(* Logix 5000 AddOnInstructionDefinition export Banner_Q5X_Jam_Param_v4; software revision 33.00; part 3 of 3 *)
(* tags used below, declared in another part *)
   Q5X : Banner_Q5X_Jam_v4;
   Port_Data : Banner_IOL_Port_v4;
   Port : DINT;
   Local_Control : DINT;
   Command_Being_Processed : BOOL;
   Update_Archive : BOOL;
   Index_Write_Inprocess : INT;
   Inprocess_Index : DINT;
(* Banner_Q5X_Jam_Param_v4, continued *)

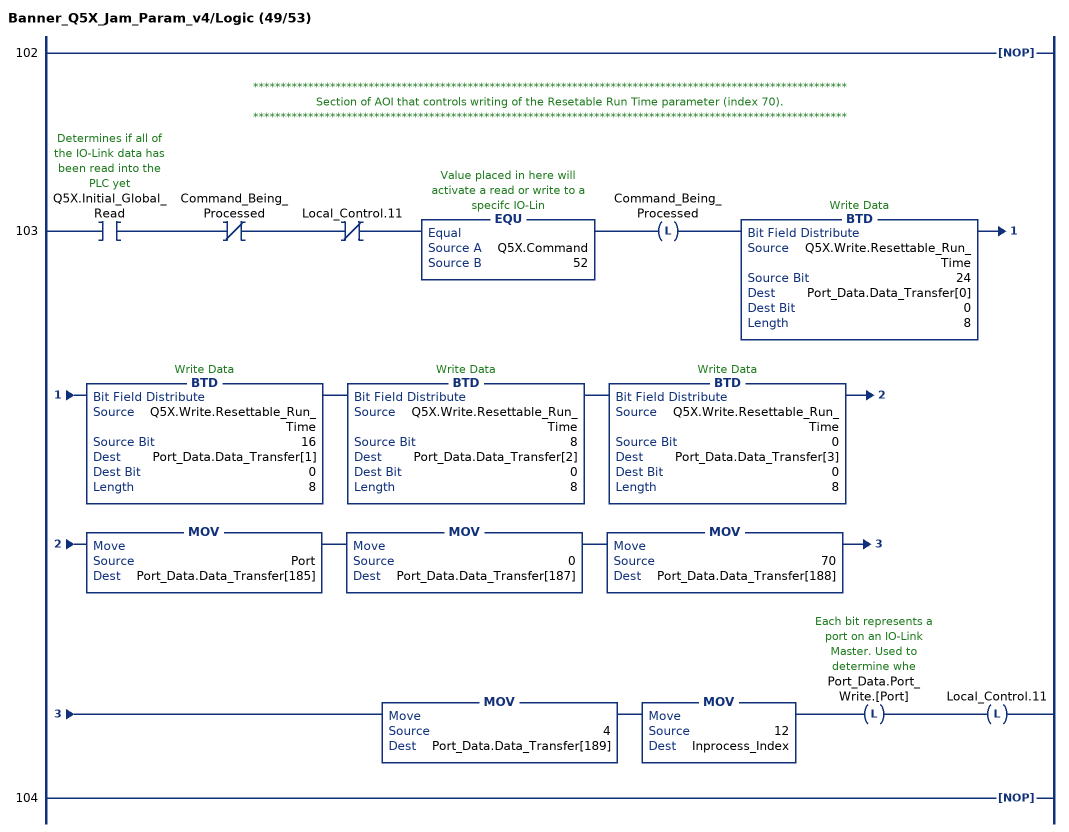
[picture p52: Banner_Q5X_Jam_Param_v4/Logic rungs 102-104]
   102: NOP();
   // ************************************************************************************************************
   // Section of AOI that controls writing of the Resetable Run Time parameter (index 70).
   // ************************************************************************************************************
   103: XIC(Q5X.Initial_Global_Read)XIO(Command_Being_Processed)XIO(Local_Control.11)EQU(Q5X.Command,52)OTL(Command_Being_Processed)BTD(Q5X.Write.Resettable_Run_Time,24,Port_Data.Data_Transfer[0],0,8)BTD(Q5X.Write.Resettable_Run_Time,16,Port_Data.Data_Transfer[1],0,8)BTD(Q5X.Write.Resettable_Run_Time,8,Port_Data.Data_Transfer[2],0,8)BTD(Q5X.Write.Resettable_Run_Time,0,Port_Data.Data_Transfer[3],0,8)MOV(Port,Port_Data.Data_Transfer[185])MOV(0,Port_Data.Data_Transfer[187])MOV(70,Port_Data.Data_Transfer[188])MOV(4,Port_Data.Data_Transfer[189])MOV(12,Inprocess_Index)OTL(Port_Data.Port_Write.[Port])OTL(Local_Control.11);
   104: NOP();
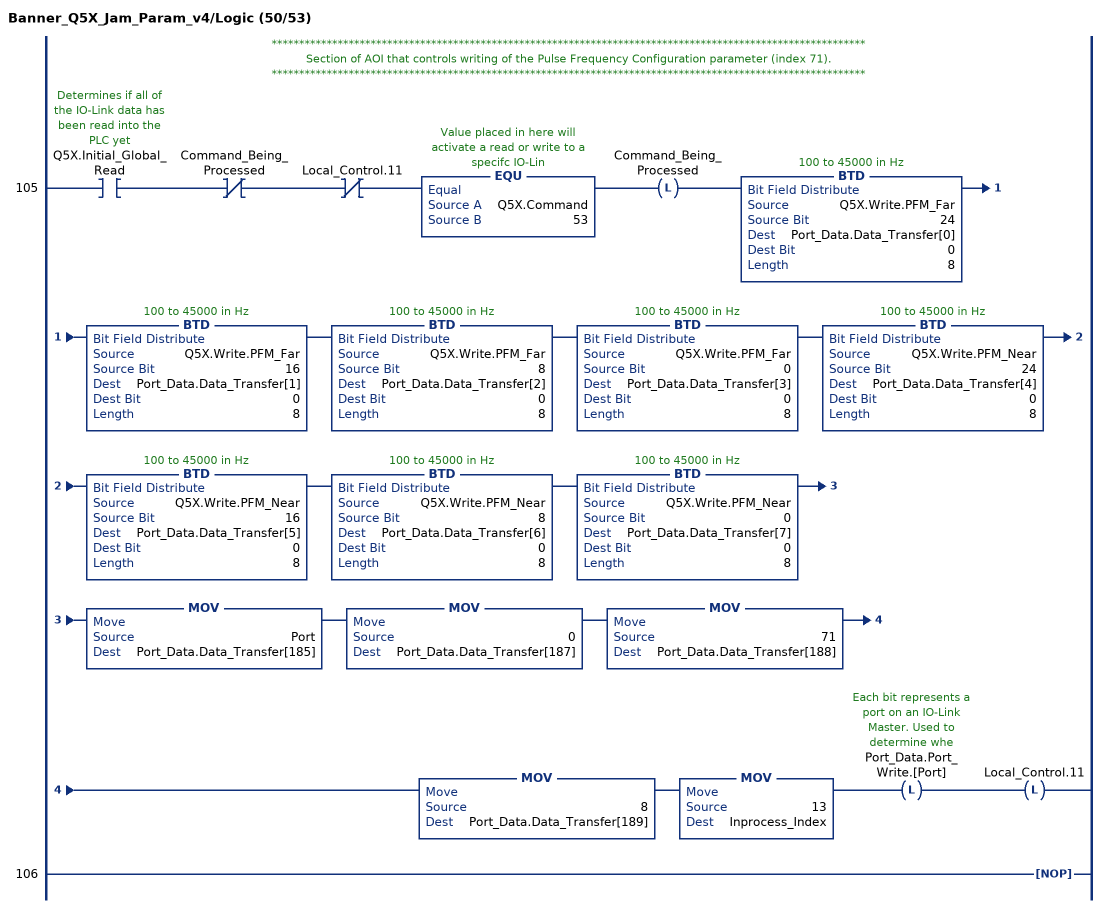
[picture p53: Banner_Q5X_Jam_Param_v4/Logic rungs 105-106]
   // ************************************************************************************************************
   // Section of AOI that controls writing of the Pulse Frequency Configuration parameter (index 71).
   // ************************************************************************************************************
   105: XIC(Q5X.Initial_Global_Read)XIO(Command_Being_Processed)XIO(Local_Control.11)EQU(Q5X.Command,53)OTL(Command_Being_Processed)BTD(Q5X.Write.PFM_Far,24,Port_Data.Data_Transfer[0],0,8)BTD(Q5X.Write.PFM_Far,16,Port_Data.Data_Transfer[1],0,8)BTD(Q5X.Write.PFM_Far,8,Port_Data.Data_Transfer[2],0,8)BTD(Q5X.Write.PFM_Far,0,Port_Data.Data_Transfer[3],0,8)BTD(Q5X.Write.PFM_Near,24,Port_Data.Data_Transfer[4],0,8)BTD(Q5X.Write.PFM_Near,16,Port_Data.Data_Transfer[5],0,8)BTD(Q5X.Write.PFM_Near,8,Port_Data.Data_Transfer[6],0,8)BTD(Q5X.Write.PFM_Near,0,Port_Data.Data_Transfer[7],0,8)MOV(Port,Port_Data.Data_Transfer[185])MOV(0,Port_Data.Data_Transfer[187])MOV(71,Port_Data.Data_Transfer[188])MOV(8,Port_Data.Data_Transfer[189])MOV(13,Inprocess_Index)OTL(Port_Data.Port_Write.[Port])OTL(Local_Control.11);
   106: NOP();
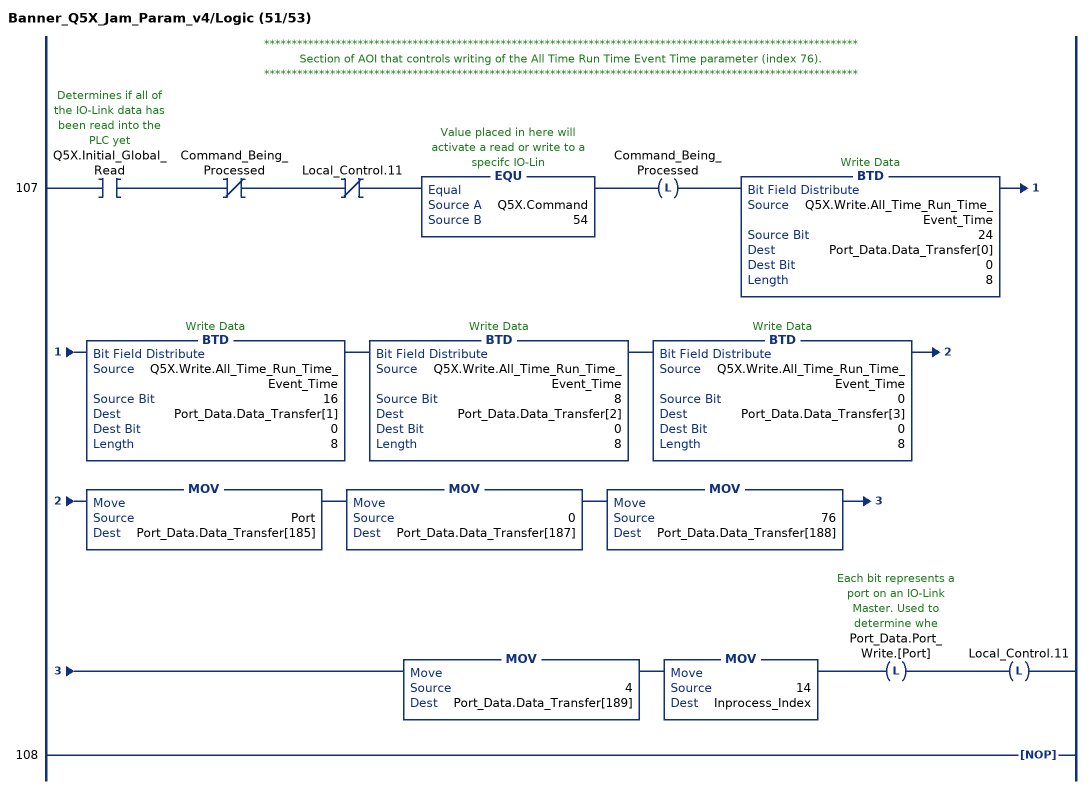
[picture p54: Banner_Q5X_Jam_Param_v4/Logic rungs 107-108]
   // ************************************************************************************************************
   // Section of AOI that controls writing of the All Time Run Time Event Time parameter (index 76).
   // ************************************************************************************************************
   107: XIC(Q5X.Initial_Global_Read)XIO(Command_Being_Processed)XIO(Local_Control.11)EQU(Q5X.Command,54)OTL(Command_Being_Processed)BTD(Q5X.Write.All_Time_Run_Time_Event_Time,24,Port_Data.Data_Transfer[0],0,8)BTD(Q5X.Write.All_Time_Run_Time_Event_Time,16,Port_Data.Data_Transfer[1],0,8)BTD(Q5X.Write.All_Time_Run_Time_Event_Time,8,Port_Data.Data_Transfer[2],0,8)BTD(Q5X.Write.All_Time_Run_Time_Event_Time,0,Port_Data.Data_Transfer[3],0,8)MOV(Port,Port_Data.Data_Transfer[185])MOV(0,Port_Data.Data_Transfer[187])MOV(76,Port_Data.Data_Transfer[188])MOV(4,Port_Data.Data_Transfer[189])MOV(14,Inprocess_Index)OTL(Port_Data.Port_Write.[Port])OTL(Local_Control.11);
   108: NOP();
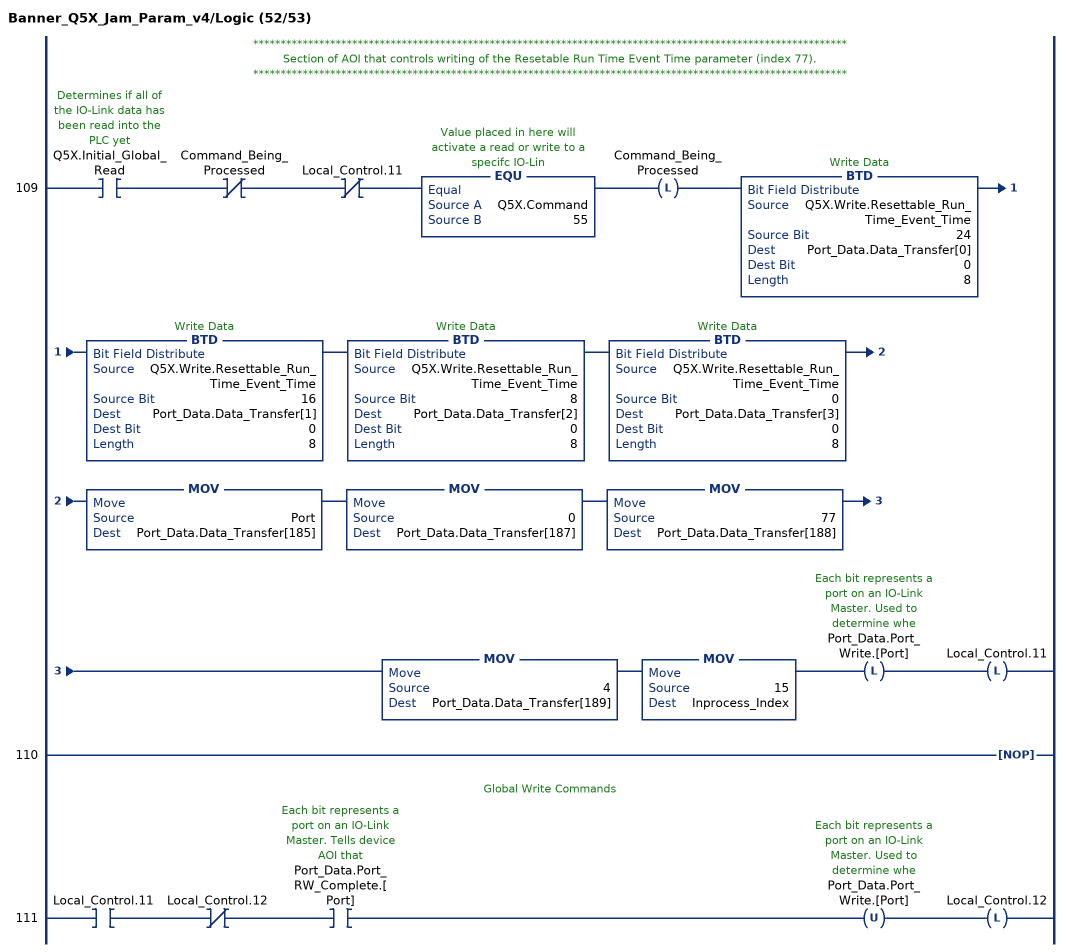
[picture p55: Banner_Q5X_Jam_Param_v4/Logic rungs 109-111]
   // ************************************************************************************************************
   // Section of AOI that controls writing of the Resetable Run Time Event Time parameter (index 77).
   // ************************************************************************************************************
   109: XIC(Q5X.Initial_Global_Read)XIO(Command_Being_Processed)XIO(Local_Control.11)EQU(Q5X.Command,55)OTL(Command_Being_Processed)BTD(Q5X.Write.Resettable_Run_Time_Event_Time,24,Port_Data.Data_Transfer[0],0,8)BTD(Q5X.Write.Resettable_Run_Time_Event_Time,16,Port_Data.Data_Transfer[1],0,8)BTD(Q5X.Write.Resettable_Run_Time_Event_Time,8,Port_Data.Data_Transfer[2],0,8)BTD(Q5X.Write.Resettable_Run_Time_Event_Time,0,Port_Data.Data_Transfer[3],0,8)MOV(Port,Port_Data.Data_Transfer[185])MOV(0,Port_Data.Data_Transfer[187])MOV(77,Port_Data.Data_Transfer[188])MOV(4,Port_Data.Data_Transfer[189])MOV(15,Inprocess_Index)OTL(Port_Data.Port_Write.[Port])OTL(Local_Control.11);
   110: NOP();
   // Global Write Commands
   111: XIC(Local_Control.11)XIO(Local_Control.12)XIC(Port_Data.Port_RW_Complete.[Port])OTU(Port_Data.Port_Write.[Port])OTL(Local_Control.12);
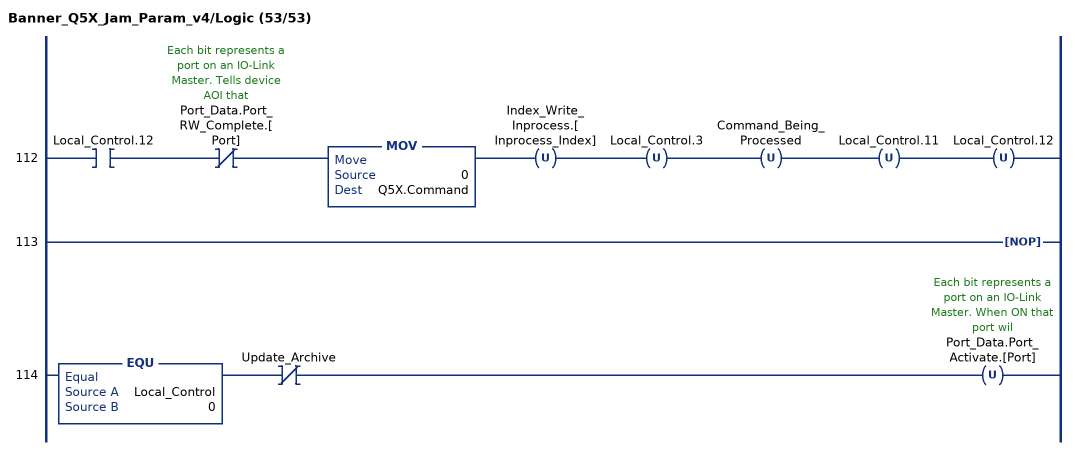
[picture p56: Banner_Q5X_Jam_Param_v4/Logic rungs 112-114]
   112: XIC(Local_Control.12)XIO(Port_Data.Port_RW_Complete.[Port])MOV(0,Q5X.Command)OTU(Index_Write_Inprocess.[Inprocess_Index])OTU(Local_Control.3)OTU(Command_Being_Processed)OTU(Local_Control.11)OTU(Local_Control.12);
   113: NOP();
   114: EQU(Local_Control,0)XIO(Update_Archive)OTU(Port_Data.Port_Activate.[Port]);
END_ROUTINE
END_ADD_ON_INSTRUCTION
